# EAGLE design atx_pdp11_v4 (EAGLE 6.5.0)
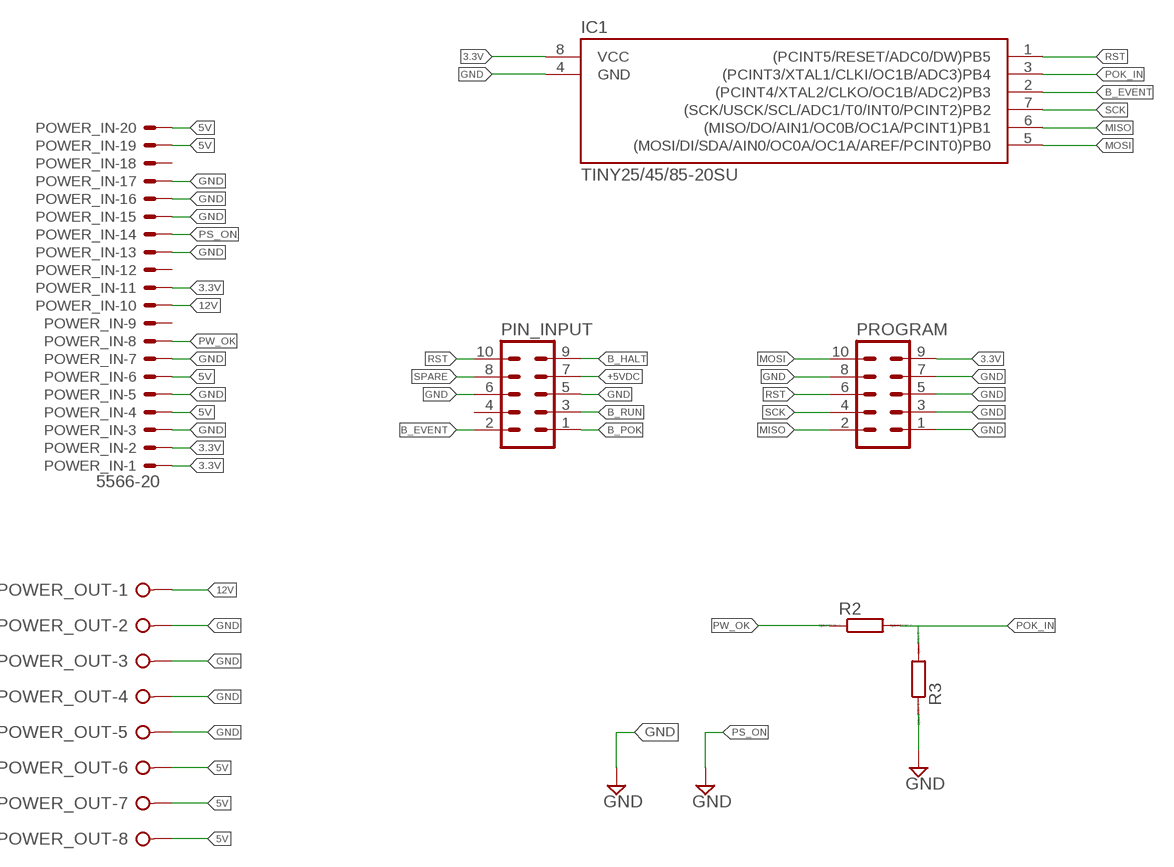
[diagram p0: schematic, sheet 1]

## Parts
IC1  TINY25/45/85-20SU  [SOIC8]
PIN_INPUT  MA05-2  [MA05-2]
POWER_IN  5566-20  [5566-20]
POWER_OUT  W237-08P  [W237-8P]
PROGRAM  MA05-2  [MA05-2]
R2  R  [R0805]
R3  R  [R0805]

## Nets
3.3V: IC1.8(VCC) POWER_IN.1 POWER_IN.2 POWER_IN.11 PROGRAM.9
5V: POWER_IN.4 POWER_IN.6 POWER_IN.19 POWER_IN.20 POWER_OUT.6 POWER_OUT.7 POWER_OUT.8
12V: POWER_IN.10 POWER_OUT.1
+5VDC: PIN_INPUT.7
B_EVENT: IC1.2((PCINT4/XTAL2/CLKO/OC1B/ADC2)PB3) PIN_INPUT.2
B_HALT: PIN_INPUT.9
B_POK: PIN_INPUT.1
B_RUN: PIN_INPUT.3
GND: IC1.4(GND) PIN_INPUT.5 PIN_INPUT.6 POWER_IN.3 POWER_IN.5 POWER_IN.7 POWER_IN.13 POWER_IN.15 POWER_IN.16 POWER_IN.17 POWER_OUT.2 POWER_OUT.3 POWER_OUT.4 POWER_OUT.5 PROGRAM.1 PROGRAM.3 PROGRAM.5 PROGRAM.7 PROGRAM.8 R3.1
MISO: IC1.6((MISO/DO/AIN1/OC0B/OC1A/PCINT1)PB1) PROGRAM.2
MOSI: IC1.5((MOSI/DI/SDA/AIN0/OC0A/OC1A/AREF/PCINT0)PB0) PROGRAM.10
POK_IN: IC1.3((PCINT3/XTAL1/CLKI/OC1B/ADC3)PB4) R2.2 R3.2
PS_ON: POWER_IN.14
PW_OK: POWER_IN.8 R2.1
RST: IC1.1((PCINT5/RESET/ADC0/DW)PB5) PIN_INPUT.10 PROGRAM.6
SCK: IC1.7((SCK/USCK/SCL/ADC1/T0/INT0/PCINT2)PB2) PROGRAM.4
SPARE: PIN_INPUT.8
Unconnected: PIN_INPUT.4 POWER_IN.9 POWER_IN.12 POWER_IN.18

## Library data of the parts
IC1 = mes_avr:TINY25/45/85: Atmel AVR ATiny25,45,85 8-bit Microcontroller
PIN_INPUT PROGRAM = con-lstb:MA05-2: PIN HEADER; OC_FARNELL: unknown; OC_NEWARK: unknown
POWER_IN = con-molex:5566-20: Mini FIT connector 20 pol ATX PC-Motherboard Power connector Source: http://www.molex.com; OC_FARNELL: unknown; OC_NEWARK: unknown
POWER_OUT = con-wago-508:W237-08P: WAGO SREW CLAMP; OC_FARNELL: unknown; OC_NEWARK: unknown
R2 R3 = eagle-ltspice:R: RESISTOR, European symbol; SPICEMODEL: NONE; SPICEPREFIX: R

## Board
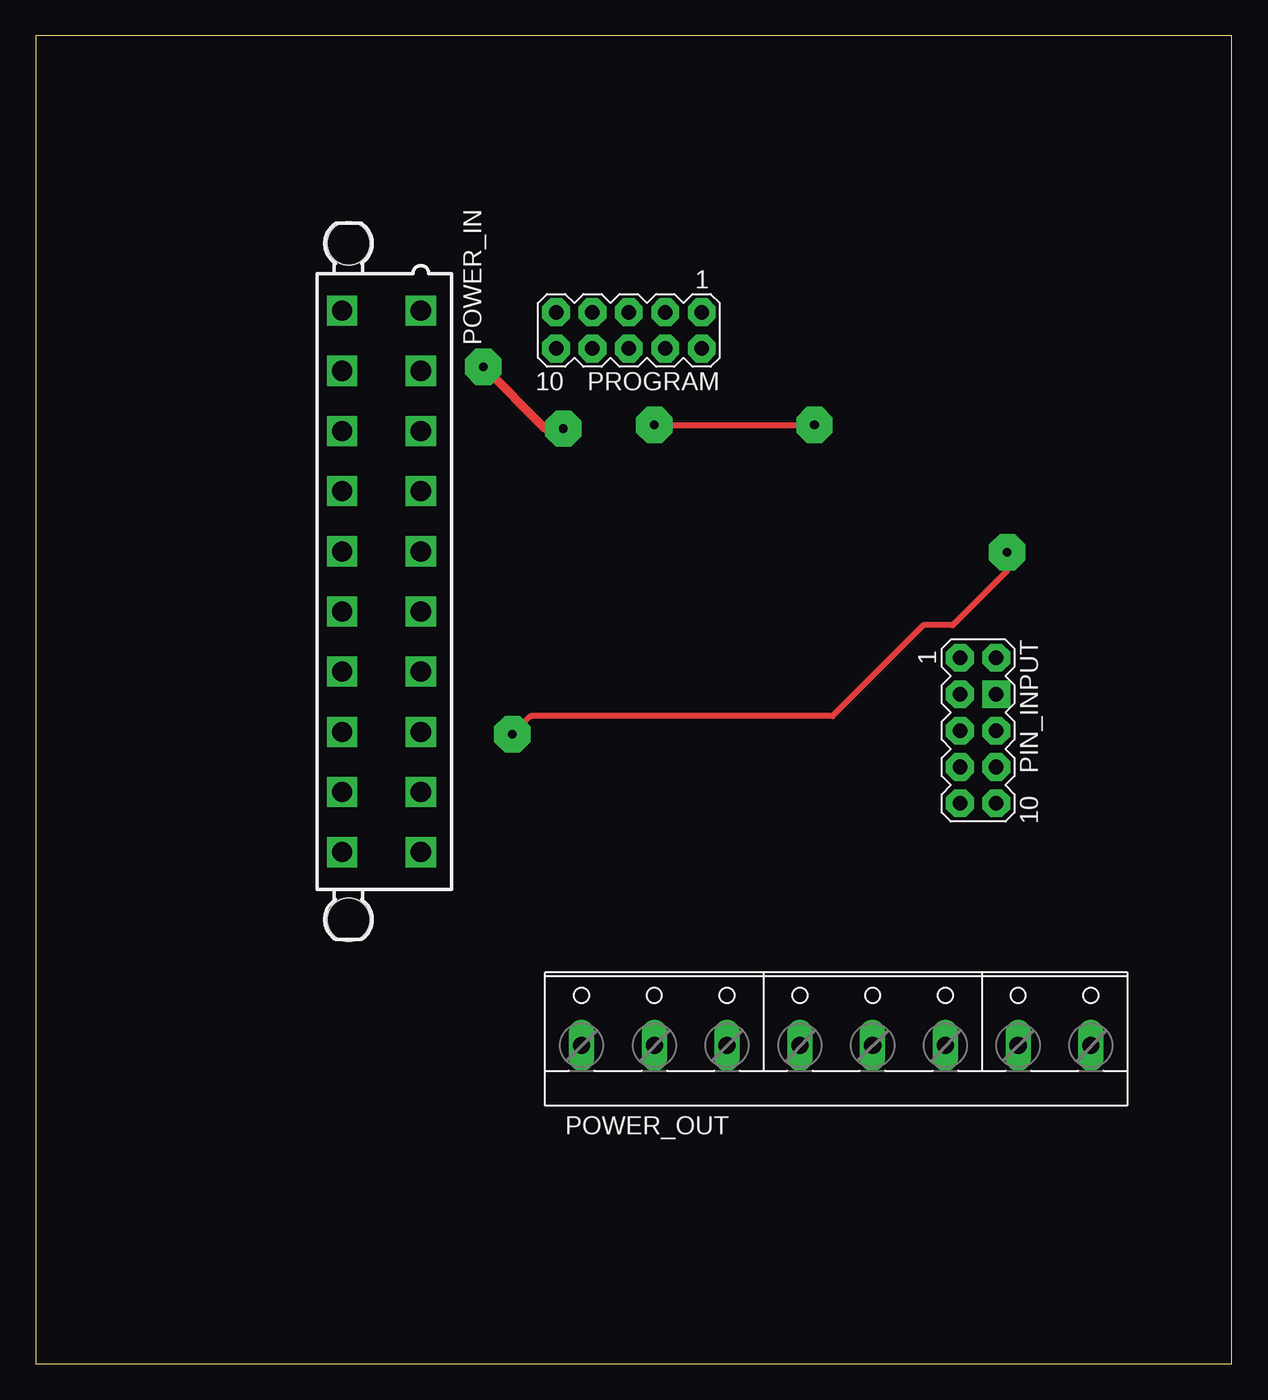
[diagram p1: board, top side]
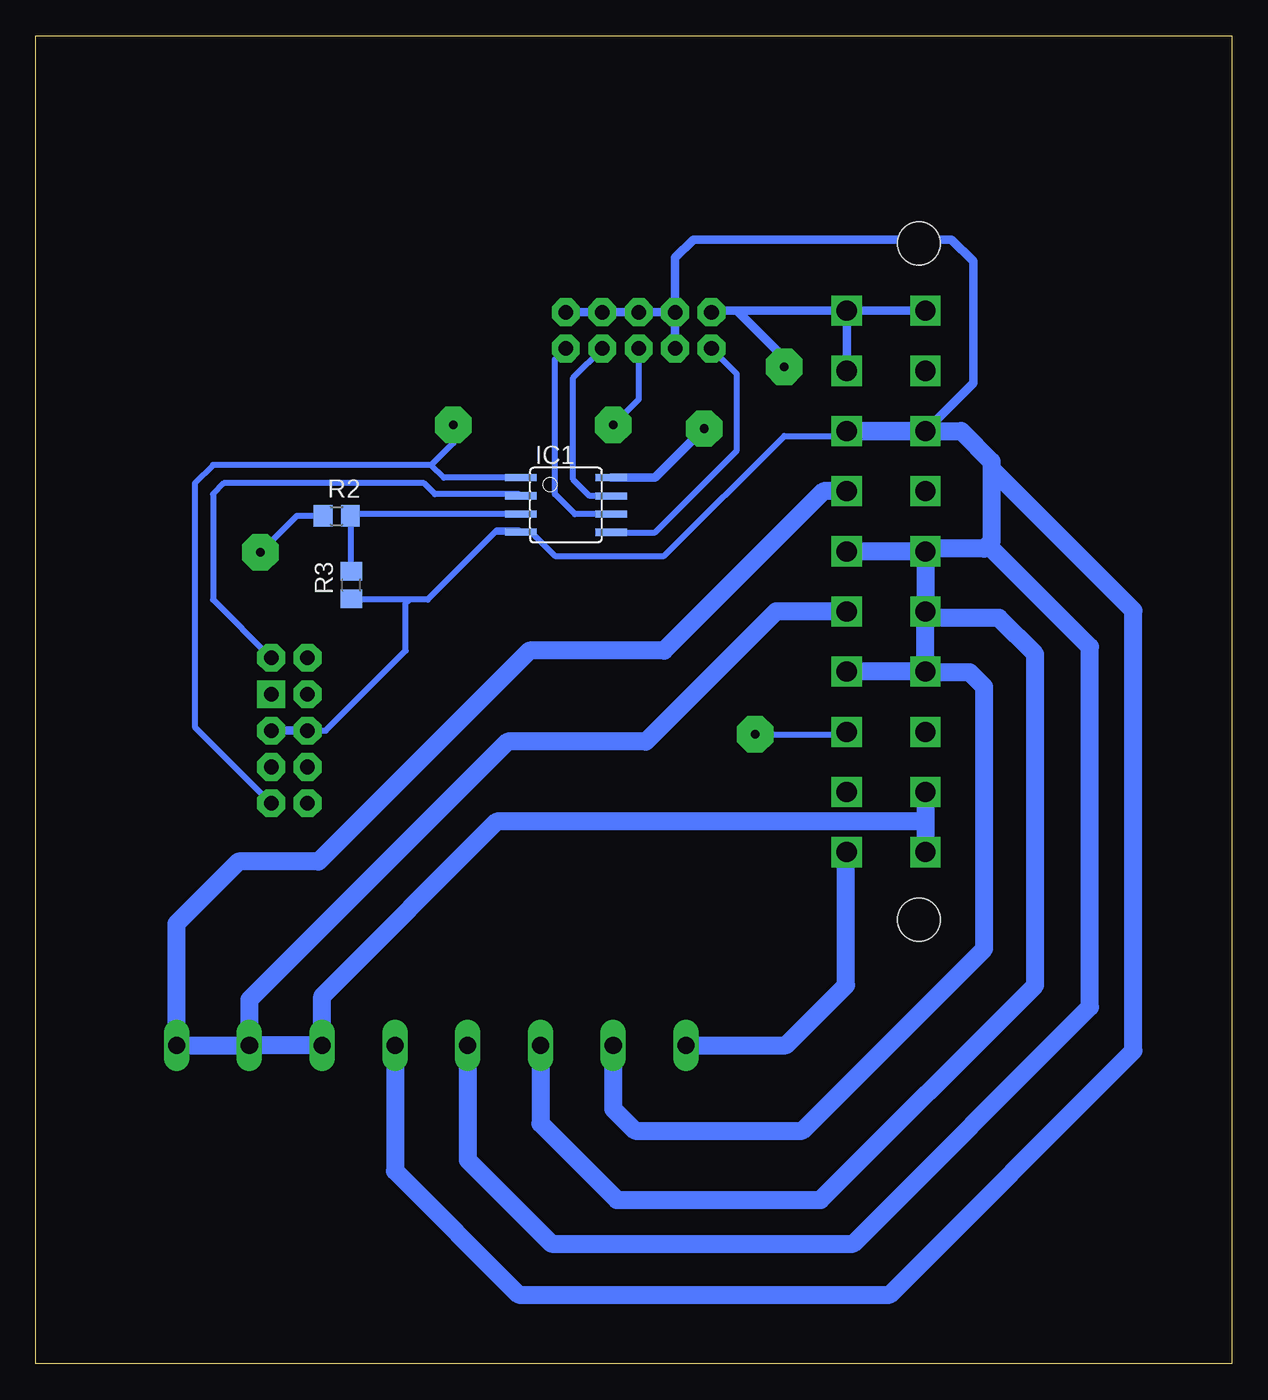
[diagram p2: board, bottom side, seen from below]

Size 83.49 x 92.7 mm. Coordinates in mm from the lower left corner, seen from the top.
Outline: 0,0 83.49,0 83.49,92.7 0,92.7 0,0
Copper layers (1*16): Top 0.035mm / dielectric 1.5mm / Bottom 0.035mm
Design rules "default": minimum track width 10mil, minimum drill 24mil, track to track 8mil, track to pad 8mil, pad to pad 8mil, via to via 8mil, smd to smd 8mil, copper to edge 40mil, drill to drill 8mil, minimum pad ring 10mil, minimum via ring 8mil, stop-mask expansion 4mil, vias tented up to drill 0mil, thermal gap 10mil

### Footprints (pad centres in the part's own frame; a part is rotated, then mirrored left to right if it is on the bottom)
SOIC8 = smd 0.5 x 2.2: 1 -1.905,-3.154; 2 -0.645,-3.154; 3 0.625,-3.154; 4 1.895,-3.154; 5 1.905,3.154; 6 0.635,3.154; 7 -0.635,3.154; 8 -1.905,3.154
MA05-2 = drill 1.016 octagon: 1 -5.08,-1.27; 2 -5.08,1.27; 3 -2.54,-1.27; 4 -2.54,1.27; 5 0,-1.27; 6 0,1.27; 7 2.54,-1.27; 8 2.54,1.27; 9 5.08,-1.27; 10 5.08,1.27
5566-20 = drill 1.4 square: 1 18.9,-2.75; 2 14.7,-2.75; 3 10.5,-2.75; 4 6.3,-2.75; 5 2.1,-2.75; 6 -2.1,-2.75; 7 -6.3,-2.75; 8 -10.5,-2.75; 9 -14.7,-2.75; 10 -18.9,-2.75; 11 18.9,2.75; 12 14.7,2.75; 13 10.5,2.75; 14 6.3,2.75; 15 2.1,2.75; 16 -2.1,2.75; 17 -6.3,2.75; 18 -10.5,2.75; 19 -14.7,2.75; 20 -18.9,2.75 | hole 3: 23.6,2.29; -23.6,2.29
W237-8P = drill 1.194 long: 1 -17.78,-0.635; 2 -12.7,-0.635; 3 -7.62,-0.635; 4 -2.54,-0.635; 5 2.54,-0.635; 6 7.62,-0.635; 7 12.7,-0.635; 8 17.78,-0.635
R0805 = smd 1.3 x 1.5: 1 -0.95,0; 2 0.95,0

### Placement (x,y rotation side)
IC1  46.48,59.94 270 bottom
PIN_INPUT  65.79,44.2 270 top
POWER_IN  24.13,54.61 90 top
POWER_OUT  55.88,22.86 0 top
PROGRAM  41.4,72.14 180 top
R2  62.48,59.18 0 bottom
R3  61.47,54.36 90 bottom

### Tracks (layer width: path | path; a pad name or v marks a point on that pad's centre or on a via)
3.3V  (via drill 0.6, 0.6 pad 1.68, 0.6 pad 2.54)
  Top 0.61: v36.83,65.28 35.56,65.28 v31.24,69.6
  Bottom 0.61: POWER_IN.2 POWER_IN.1 POWER_IN.11 34.54,73.51 | 34.54,73.51 36.22,73.51 PROGRAM.9 | IC1.8 40.26,61.85 v36.83,65.28 | v31.24,69.6 31.24,70.21 34.54,73.51
5V
  Bottom 1.27: POWER_IN.20 POWER_IN.19 21.38,38.06 21.59,37.85 51.31,37.85 63.5,25.65 POWER_OUT.6 POWER_OUT.7 | POWER_IN.4 28.5,60.91 39.62,49.78 49.02,49.78 63.75,35.05 69.34,35.05 73.66,30.73 POWER_OUT.8 POWER_OUT.7 | POWER_IN.6 31.82,52.51 40.89,43.43 50.55,43.43 68.58,25.4 POWER_OUT.7
12V
  Bottom 1.27: POWER_OUT.1 31.11,22.23 26.92,26.42 26.92,35.67 POWER_IN.10
B_EVENT
  Bottom 0.406: IC1.2 49.75,60.71 55.63,60.71 56.39,61.47 70.36,61.47 71.12,60.71 71.12,53.34 PIN_INPUT.2
GND
  Bottom 0.406: IC1.4 51.42,58.05 | 51.42,58.05 56.13,53.34 57.4,53.34 | 57.4,53.34 57.66,53.34 | 57.66,53.34 61.4,53.34 R3.1 | PIN_INPUT.5 63.25,44.2 57.66,49.78 57.66,53.09 | 57.66,53.09 57.4,53.34 | IC1.4 49.67,58.05 49.78,58.17 51.31,58.17 51.42,58.05 | 57.66,53.34 57.66,53.09 | POWER_IN.3 27.22,64.77 31.24,64.77 39.62,56.39 47.24,56.39 48.91,58.05 IC1.4
  Bottom 0.61: PIN_INPUT.6 PIN_INPUT.5 | PROGRAM.1 PROGRAM.3 PROGRAM.5 PROGRAM.7 PROGRAM.8 38.86,77.22 37.59,78.49 19.56,78.49 18.03,76.96 18.03,68.46 POWER_IN.13
  Bottom 1.27: POWER_IN.13 POWER_IN.3 18.88,65.11 16.76,62.99 16.76,62.48 | 22.1,56.71 POWER_IN.15 POWER_IN.16 | 22.1,56.71 POWER_IN.5 | POWER_IN.17 POWER_IN.7 | POWER_IN.17 POWER_IN.16 | 16.76,62.48 16.76,57.4 17.02,57.15 | 17.02,57.15 17.27,56.9 21.91,56.9 22.1,56.71 | POWER_OUT.2 43.18,17.78 41.66,16.26 29.97,16.26 17.27,28.96 17.27,47.24 18.29,48.26 21.33,48.26 POWER_IN.17 | POWER_OUT.3 48.26,16.76 42.93,11.43 28.7,11.43 13.72,26.42 13.72,49.53 16.26,52.07 20.94,52.07 POWER_IN.16 | POWER_OUT.4 53.34,14.22 47.5,8.38 26.42,8.38 9.91,24.89 9.91,50.04 17.02,57.15 | POWER_OUT.5 58.42,13.46 49.78,4.83 23.88,4.83 6.86,21.84 6.86,52.58 16.76,62.48
MISO
  Bottom 0.406: IC1.6 45.85,59.31 47.24,60.71 47.24,70.1 PROGRAM.2
MOSI
  Bottom 0.406: IC1.5 40.26,58.04 34.54,63.75 34.54,69.09 35.94,70.48
  Bottom 0.61: 35.94,70.48 PROGRAM.10
N$1  (via drill 0.6 pad 1.68)
  other vias: 67.06,46.74
N$2  (via drill 0.6 pad 1.93)
  other vias: 67.06,46.74
N$3  (via drill 0.6 pad 1.93)
  other vias: 64.52,49.28
N$4  (via drill 0.6 pad 1.93)
  other vias: 64.52,46.74
N$5  (via drill 0.6 pad 1.93)
  other vias: 64.52,44.2
N$6  (via drill 0.6 pad 1.93)
  other vias: 64.52,41.66
N$7  (via drill 0.8 pad 1.68)
  other vias: 67.06,49.28
N$8  (via drill 0.8 pad 1.68)
  other vias: 67.06,44.2
N$9  (via drill 0.8 pad 1.68)
  other vias: 64.52,44.2
N$10  (via drill 0.8 pad 1.68)
  other vias: 64.52,46.74
N$11  (via drill 0.8 pad 1.68)
  other vias: 64.52,49.28
N$12  (via drill 0.6 pad 1.93)
  other vias: 67.06,39.12
N$13  (via drill 0.6 pad 1.93)
  other vias: 64.52,39.12
N$14  (via drill 0.6 pad 1.93)
  other vias: 67.06,41.66
N$15  (via drill 0.6 pad 1.93)
  other vias: 67.06,44.2
N$16  (via drill 0.8 pad 1.68)
  other vias: 67.06,39.12
N$17  (via drill 0.8 pad 1.68)
  other vias: 67.06,41.66
N$18  (via drill 0.8 pad 1.68)
  other vias: 64.52,41.66
N$19  (via drill 0.8 pad 1.68)
  other vias: 64.52,39.12
N$20  (via drill 0.8 pad 1.68)
  other vias: 64.52,44.2
N$21  (via drill 0.8 pad 1.68)
  other vias: 36.32,70.87
N$22  (via drill 0.8 pad 1.68)
  other vias: 38.86,70.87
N$23  (via drill 0.8 pad 1.68)
  other vias: 41.4,70.87
N$24  (via drill 0.8 pad 1.68)
  other vias: 43.94,70.87
N$25  (via drill 0.8 pad 1.68)
  other vias: 46.48,73.41
N$26  (via drill 0.8 pad 1.68)
  other vias: 46.48,70.87
N$27  (via drill 0.8 pad 1.68)
  other vias: 43.94,73.41
N$28  (via drill 0.6 pad 1.93)
  other vias: 67.06,49.28
N$29  (via drill 0.6 pad 1.93)
  other vias: 36.32,73.41
N$30  (via drill 0.8 pad 1.68)
  other vias: 41.4,73.41
N$31  (via drill 0.8 pad 1.68)
  other vias: 36.32,73.41
N$32  (via drill 0.8 pad 1.68)
  other vias: 38.86,73.41
N$33  (via drill 0.6 pad 1.93)
  other vias: 36.32,70.87
N$34  (via drill 0.6 pad 1.93)
  other vias: 38.86,70.87
N$35  (via drill 0.6 pad 1.93)
  other vias: 41.4,70.87
N$36  (via drill 0.6 pad 1.93)
  other vias: 43.94,70.87
N$37  (via drill 0.6 pad 1.93)
  other vias: 46.48,70.87
N$38  (via drill 0.6 pad 1.93)
  other vias: 43.94,73.41
N$39  (via drill 0.6 pad 1.93)
  other vias: 41.4,73.41
N$40  (via drill 0.6 pad 1.93)
  other vias: 38.86,73.41
N$41  (via drill 0.6 pad 1.93)
  other vias: 46.48,73.41
POK_IN
  Bottom 0.406: IC1.3 61.4,59.32 R2.2 61.47,59.12 R3.2
PW_OK  (via drill 0.6, 0.6 pad 1.68, 0.6 pad 2.54)
  Top 0.406: v67.82,56.64 67.82,55.37 64.01,51.56 61.98,51.56 55.63,45.21 34.54,45.21 v33.27,43.94
  Bottom 0.406: R2.1 65.28,59.18 v67.82,56.64 | v33.27,43.94 27.05,43.94 POWER_IN.8
RST  (via drill 0.6, 0.6 pad 1.68, 0.6 pad 2.54)
  Top 0.406: v43.18,65.53 v54.36,65.53
  Bottom 0.406: IC1.1 54.99,61.85 55.88,62.74 | 55.88,62.74 71.12,62.74 72.39,61.47 72.39,44.45 PIN_INPUT.10 | PROGRAM.6 41.4,67.31 v43.18,65.53 | v54.36,65.53 54.36,64.26 55.88,62.74
SCK
  Bottom 0.406: IC1.7 44.83,60.58 45.97,61.72 45.97,68.83 PROGRAM.4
